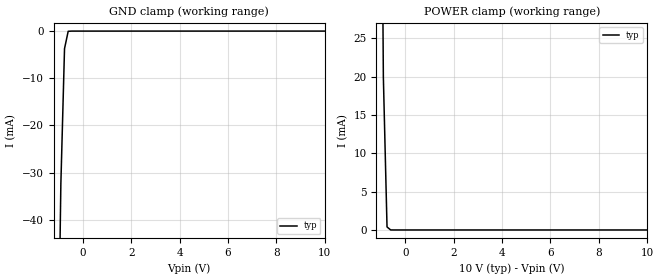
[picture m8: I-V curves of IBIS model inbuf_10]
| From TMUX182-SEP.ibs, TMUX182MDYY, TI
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| inbuf_10
[Model]   inbuf_10
Model_type   Input
Vinl = 0.8
Vinh = 1.35
|   typ   min   max
C_comp   6.362683e-13   NA   NA
[Voltage Range]   10   NA   NA
[Temperature Range]   27   NA   NA
[Power Clamp Reference]   10   NA   NA
[GND Clamp Reference]   0   NA   NA
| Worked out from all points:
|   GND clamp passes 1 mA (typ) near -0.65 V on its own axis
|   POWER clamp passes 1 mA (typ) near -0.76 V on its own axis
[GND Clamp]
|   Voltage   I(typ)   I(min)   I(max)
-5V       -2.674A    NA         NA
-1.061V   -87.09mA   NA         NA
-909.1mV  -32.43mA   NA         NA
-757.6mV  -3.722mA   NA         NA
-606.1mV  -41.61uA   NA         NA
10V       464.8nA    NA         NA
[POWER Clamp]
|   Voltage   I(typ)   I(min)   I(max)
-5V       3.29A      NA         NA
-1.061V   85.94mA    NA         NA
-909.1mV  19.94mA    NA         NA
-757.6mV  394.2uA    NA         NA
-606.1mV  1.999uA    NA         NA
10V       -13.44pA   NA         NA
